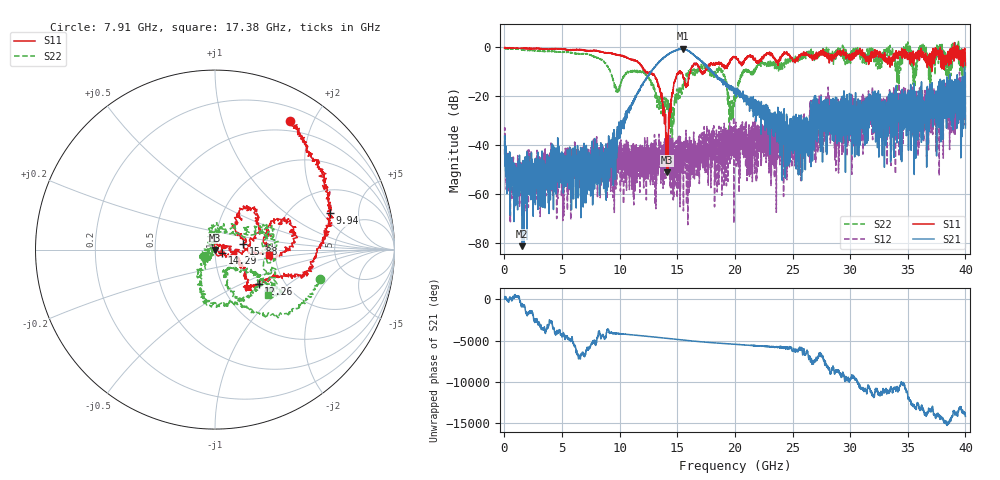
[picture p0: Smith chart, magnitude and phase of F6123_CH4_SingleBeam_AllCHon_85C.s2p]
!Keysight Technologies,N5245B,MY55451909,A.17.20.08
!Date: Wednesday, November 22, 2023 09:47:29
!Correction: S11(C  2-Port  )
!S21(C  2-Port  )
!S12(C  2-Port  )
!S22(C  2-Port  )
!S2P File: Measurements: S11, S21, S12, S22:
# Hz S  RI  R 50
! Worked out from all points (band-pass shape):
!   4000 points, 10 MHz to 40 GHz, reference 50 ohm
!   highest |S21| = -0.82 dB at 15.51 GHz (marker M1); lowest = -81.2 dB at 1.55 GHz (marker M2)
!   |S21| within 3 dB of the highest: 13.99317 GHz to 14.02981 GHz (36.63 MHz wide, 0.261 % of centre); 14.03 GHz to 16.5 GHz (2.467 GHz wide, 16.2 % of centre)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
!   lowest |S11| = -51.2 dB at 14.09 GHz (marker M3), VSWR 1.01, Z = 49.8 - j0.179 ohm
!   |S11| at or under -10 dB: 12.21 GHz to 15.18 GHz (2.965 GHz wide, 21.7 % of centre); 15.24 GHz to 16.14 GHz (897.4 MHz wide, 5.72 % of centre); 17.08 GHz to 17.28 GHz (195.9 MHz wide, 1.14 % of centre)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
!   |S22| runs from -52.3 to 2.5 dB; largest |S21 - S12| = 0.91
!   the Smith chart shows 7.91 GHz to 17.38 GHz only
!   S11 on the Smith chart (normalised r, x): 7.91 GHz: 0.37, +1.68; 9.94 GHz: 3.22, +2.36; 12.26 GHz: 1.49, -0.62; 14.29 GHz: 1.08, -0.04; 15.88 GHz: 1.37, +0.08; 17.38 GHz: 1.85, -0.12
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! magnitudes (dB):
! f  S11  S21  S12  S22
! 10 MHz  -0.5  -40.1  -43.9  -1.0
! 1.55 GHz  -0.6  -81.2  -47.6  -1.3
! 6.68 GHz  -1.3  -62.6  -45.8  -2.8
! 7.91 GHz  -1.6  -48.9  -42.6  -4.3
! 8.78 GHz  -2.4  -56.2  -46.4  -6.6
! 9.94 GHz  -3.5  -32.6  -46.8  -16.6
! 12.26 GHz  -10.2  -13.1  -44.6  -11.0
! 13.34 GHz  -14.9  -6.6  -43.2  -22.2
! 14.09 GHz  -51.2  -3.5  -40.0  -26.2
! 14.29 GHz  -27.2  -2.9  -40.6  -29.7
! 14.85 GHz  -13.3  -1.6  -42.2  -19.8
! 15.51 GHz  -12.1  -0.8  -51.3  -16.8
! 15.88 GHz  -15.9  -1.6  -37.7  -11.8
! 17.38 GHz  -10.4  -7.3  -44.1  -8.1
! 20.01 GHz  -4.4  -17.8  -35.5  -20.9
! 20.82 GHz  -5.5  -21.4  -38.3  -9.2
! 24.56 GHz  -3.3  -35.3  -32.0  -4.9
! 26.67 GHz  -3.7  -26.0  -27.1  -2.8
! 33.34 GHz  -5.4  -25.9  -32.2  -1.1
! 35.6 GHz  -4.7  -31.1  -31.4  -15.8
! 39.26 GHz  -1.7  -17.7  -16.2  -0.7
! 40 GHz  -7.6  -33.1  -32.1  -9.3
